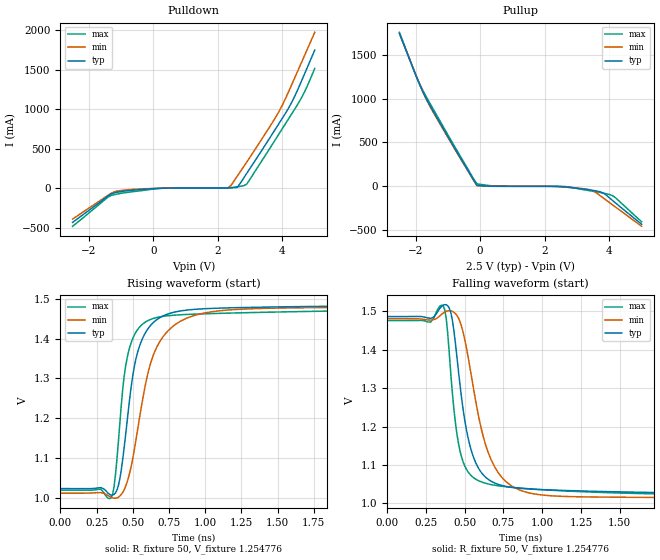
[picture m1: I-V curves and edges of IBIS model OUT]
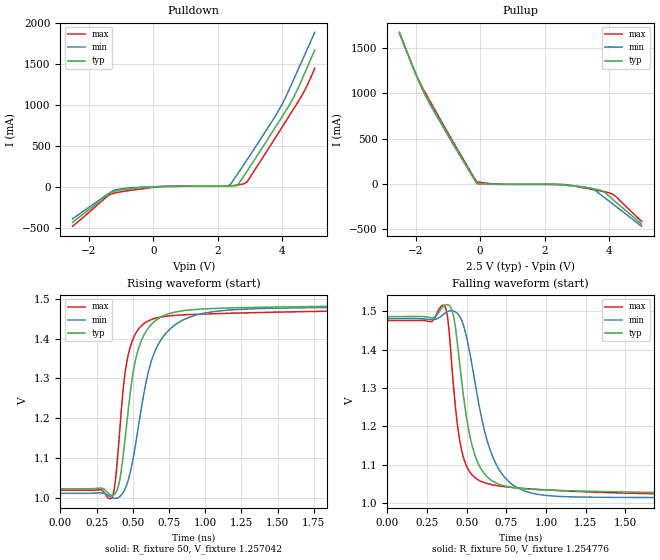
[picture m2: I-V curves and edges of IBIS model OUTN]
|   IBIS File of SG2520VGN D
|   LVDS, Vcc=2.5V, Io=4.5mA, fo>212.5MHz
[IBIS Ver]   3.2
[File Name]   sg2520vgn_hf_45m_25v.ibs
[File Rev]   1.0
[Date]   July 24, 2020
[Source]
Fairchild Ensigna Lab's Method
[Notes]
Created by Minoru Kozaki
[Disclaimer]
Seiko Epson Corporation makes no warranty with respect to the
information contained herein.
[Copyright]
Copyright(C) 2020, Seiko Epson Corporation. All rights reserved.
|   Component
[Component]   SG2520VGN
[Manufacturer]  Seiko Epson Corporation
[Package]
R_pkg   17.7m   NA   NA
L_pkg   235p   NA   NA
C_pkg   208f   NA   NA
[Pin]   signal_name   model_name   R_pin   L_pin   C_pin
1   OE/ST   NC
2   NC   NC
3   GND   GND
4   OUT   OUT   17.7m   235p   208f
5   OUTN   OUTN   10.4m   129p   221f
6   VCC   POWER
[Diff Pin] inv_pin  vdiff  tdelay_typ
4   5   0   0
| Models and submodels in the file (2): OUT (Output), OUTN (Output)
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|   Model OUT
[Model]   OUT
Model_type   Output
Polarity   Non-Inverting
Vref = 1.25
Vmeas = 1.25
Rref = 50
Cref = 0
C_comp   4.5p   4.5p   4.5p
[Temperature Range]   25   105   -40
[Voltage Range]   2.5   2.25   2.75
[Pullup Reference]   2.5   2.25   2.75
[Pulldown Reference]   0   0   0
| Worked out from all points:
|   slope of the pulldown table from 0 to 0.375 V, typ, clamps not added: 59.2 ohm
|   slope of the pullup table from 0 to 0.375 V, typ, clamps not added: 50.4 ohm
|   falling waveform, R_fixture 50, V_fixture 1.254776: 20-80 % time 114ps typ, 160ps min, 85.9ps max; typ from 1.49 V to 1.02 V
|   rising waveform, R_fixture 50, V_fixture 1.254776: 20-80 % time 122ps typ, 174ps min, 90ps max; typ from 1.02 V to 1.49 V
[Pullup]
-2.5V     1.749A     1.743A     1.76A
-2V       1.273A     1.28A      1.276A
-1.8V     1.098A     1.1A       1.112A
-1.6V     952.7mA    943.3mA    976mA
-800mV    439.2mA    429.8mA    457.1mA
-100mV    7.193mA    2.17mA     24.05mA
500mV     -4.416mA   -4.533mA   -3.19mA
2.6V      -12.42mA   -12.9mA    -6.607mA
3.4V      -46.01mA   -45.23mA   -55.59mA
3.8V      -79.93mA   -135.8mA   -81.97mA
4.1V      -167.3mA   -217.6mA   -112.2mA
5V        -439.5mA   -463.2mA   -411.3mA
[Pulldown]
-2.5V     -430.6mA   -388.6mA   -480mA
-1.4V     -95.36mA   -87.03mA   -110.1mA
-1.2V     -55.06mA   -42.56mA   -78.4mA
200mV     672.5uA    1.166mA    -333.1uA
2.3V      5.906mA    5.681mA    6.825mA
2.4V      6.817mA    33.73mA    9.538mA
2.6V      12.6mA     154.3mA    19.88mA
2.9V      194mA      337mA      56.62mA
3.9V      826.3mA    978.8mA    694.8mA
4.3V      1.1A       1.326A     952.2mA
4.6V      1.37A      1.604A     1.155A
5V        1.751A     1.976A     1.519A
[Falling Waveform]
R_fixture = 50
V_fixture = 1.254776
V_fixture_min = 1.245697
V_fixture_max = 1.248050
0s        1.486V     1.48V      1.476V
280ps     1.481V     1.477V     1.471V
350ps     1.512V     1.491V     1.516V
390ps     1.514V     1.501V     1.442V
440ps     1.415V     1.494V     1.208V
490ps     1.242V     1.444V     1.107V
580ps     1.098V     1.245V     1.061V
730ps     1.048V     1.072V     1.045V
1.1ns     1.034V     1.019V     1.033V
4ns       1.024V     1.012V     1.02V
[Rising Waveform]
R_fixture = 50
V_fixture = 1.254776
V_fixture_min = 1.245697
V_fixture_max = 1.248050
0s        1.024V     1.012V     1.02V
340ps     1.009V     1.004V     998.2mV
380ps     1.013V     999.3mV    1.058V
430ps     1.097V     1.014V     1.273V
470ps     1.223V     1.051V     1.367V
530ps     1.362V     1.165V     1.421V
640ps     1.44V      1.357V     1.45V
800ps     1.467V     1.437V     1.459V
1.1ns     1.477V     1.47V      1.463V
4ns       1.485V     1.48V      1.475V
[Ramp]
R_load = 50
dV/dt_r   0.27837/122.97p   0.28188/174.64p   0.27465/90.98p
dV/dt_f   0.27837/114.68p   0.28188/161.50p   0.27465/86.20p
|   Model OUTN
[Model]   OUTN
Model_type   Output
Polarity   Inverting
Vref = 1.25
Vmeas = 1.25
Rref = 50
Cref = 0
C_comp   4.5p   4.5p   4.5p
[Temperature Range]   25   105   -40
[Voltage Range]   2.5   2.25   2.75
[Pullup Reference]   2.5   2.25   2.75
[Pulldown Reference]   0   0   0
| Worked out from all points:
|   slope of the pulldown table from 0 to 0.375 V, typ, clamps not added: 59.2 ohm
|   slope of the pullup table from 0 to 0.375 V, typ, clamps not added: 50.5 ohm
|   falling waveform, R_fixture 50, V_fixture 1.254776: 20-80 % time 112ps typ, 159ps min, 84.7ps max; typ from 1.49 V to 1.02 V
|   rising waveform, R_fixture 50, V_fixture 1.257042: 20-80 % time 121ps typ, 172ps min, 89.8ps max; typ from 1.02 V to 1.49 V
[Pullup]
-2.5V     1.664A     1.661A     1.673A
-2V       1.214A     1.22A      1.219A
-1.7V     983.7mA    977.2mA    1.005A
-1V       546.3mA    536.3mA    564.6mA
-100mV    7.191mA    2.172mA    24.01mA
500mV     -4.416mA   -4.534mA   -3.192mA
2.6V      -12.44mA   -13.04mA   -6.609mA
3.4V      -46.55mA   -45.7mA    -55.96mA
3.6V      -59.07mA   -81.01mA   -68.58mA
3.8V      -80.48mA   -136.7mA   -82.74mA
4.1V      -168.4mA   -219.2mA   -112.8mA
5V        -443.2mA   -467.7mA   -413.7mA
[Pulldown]
-2.5V     -434.7mA   -392.5mA   -483.9mA
-1.4V     -96.19mA   -87.87mA   -110.7mA
-1.2V     -55.54mA   -42.93mA   -78.98mA
200mV     671.6uA    1.167mA    -336.9uA
2.3V      5.907mA    5.681mA    6.826mA
2.4V      6.815mA    32.6mA     9.531mA
2.6V      12.59mA    149mA      19.84mA
2.9V      187.3mA    325.3mA    54.87mA
4V        859.3mA    1.013A     732.9mA
4.4V      1.133A     1.352A     981.5mA
4.7V      1.394A     1.617A     1.183A
5V        1.666A     1.882A     1.444A
[Falling Waveform]
R_fixture = 50
V_fixture = 1.254776
V_fixture_min = 1.245697
V_fixture_max = 1.248050
0s        1.486V     1.48V      1.475V
280ps     1.482V     1.478V     1.473V
360ps     1.515V     1.494V     1.514V
400ps     1.51V      1.501V     1.395V
440ps     1.423V     1.495V     1.211V
490ps     1.249V     1.449V     1.107V
580ps     1.098V     1.252V     1.06V
730ps     1.046V     1.073V     1.044V
1.1ns     1.033V     1.018V     1.033V
4ns       1.024V     1.012V     1.02V
[Rising Waveform]
R_fixture = 50
V_fixture = 1.257042
V_fixture_min = 1.247965
V_fixture_max = 1.250296
0s        1.023V     1.012V     1.02V
340ps     1.009V     1.005V     998.4mV
380ps     1.012V     999.3mV    1.045V
430ps     1.097V     1.012V     1.261V
470ps     1.226V     1.047V     1.362V
530ps     1.364V     1.16V      1.419V
640ps     1.44V      1.357V     1.449V
800ps     1.467V     1.437V     1.458V
1.1ns     1.476V     1.469V     1.463V
4ns       1.485V     1.48V      1.475V
[Ramp]
R_load = 50
dV/dt_r   0.27808/121.55p   0.28160/172.44p   0.27436/90.81p
dV/dt_f   0.27808/112.85p   0.28160/160.06p   0.27436/84.66p
